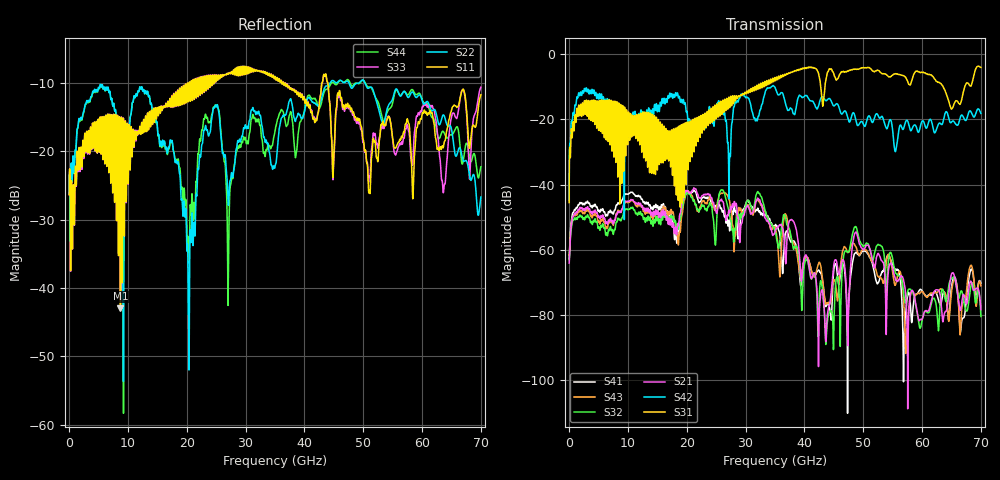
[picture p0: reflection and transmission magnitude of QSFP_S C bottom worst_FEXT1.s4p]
! AWR Design Environment (8415) Tue Jan 08 12:50:50 2019
! Document = 'QSFP Channel_S'
! nPorts: 4, nXvals: 7001
# HZ S DB R 50
!Freq DBS11 AngS11 DBS12 AngS12 DBS13 AngS13 DBS14 AngS14
!	DBS21 AngS21 DBS22 AngS22 DBS23 AngS23 DBS24 AngS24
!	DBS31 AngS31 DBS32 AngS32 DBS33 AngS33 DBS34 AngS34
!	DBS41 AngS41 DBS42 AngS42 DBS43 AngS43 DBS44 AngS44
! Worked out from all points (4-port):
!   7000 points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, 10 MHz to 70 GHz, reference 50 ohm
!   strongest paths, dB at 10 MHz, 17.51 GHz, 35.01 GHz, 52.51 GHz, 70 GHz:
!     S31: -45.5, -26.4, -7.4, -5.0, -4.0
!     S42: -44.8, -12.5, -10.2, -18.8, -18.2
!     S21: -64.1, -52.8, -54.4, -61.2, -78.4
!     S32: -63.1, -50.6, -54.4, -58.4, -80.5
!     S43: -61.7, -48.8, -53.1, -68.2, -71.1
!     S41: -62.7, -51.4, -52.7, -70.3, -70.3
!   lowest |S11| = -43.0 dB at 8.74 GHz (marker M1), VSWR 1.01, Z = 50.7 + j0.249 ohm
!   |S11| at or under -10 dB: start of sweep to 20.44 GHz; 36.44 GHz to 43.03 GHz (6.585 GHz wide, 16.6 % of centre); 43.97 GHz to end of sweep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
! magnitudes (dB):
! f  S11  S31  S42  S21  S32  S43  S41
! 10 MHz  -26.4  -45.5  -44.8  -64.1  -63.1  -61.7  -62.7
! 2.63 GHz  -18.1  -14.4  -10.5  -48.0  -50.8  -49.0  -46.2
! 8.74 GHz  -43.0  -16.2  -27.0  -48.5  -51.0  -48.4  -45.8
! 32.21 GHz  -8.3  -9.6  -19.0  -44.7  -42.6  -45.1  -48.2
! 44.34 GHz  -13.1  -4.5  -13.7  -76.4  -79.0  -76.6  -78.5
! 48.65 GHz  -15.0  -4.5  -19.5  -54.7  -52.9  -58.9  -61.0
! 70 GHz  -11.8  -4.0  -18.2  -78.4  -80.5  -71.1  -70.3
